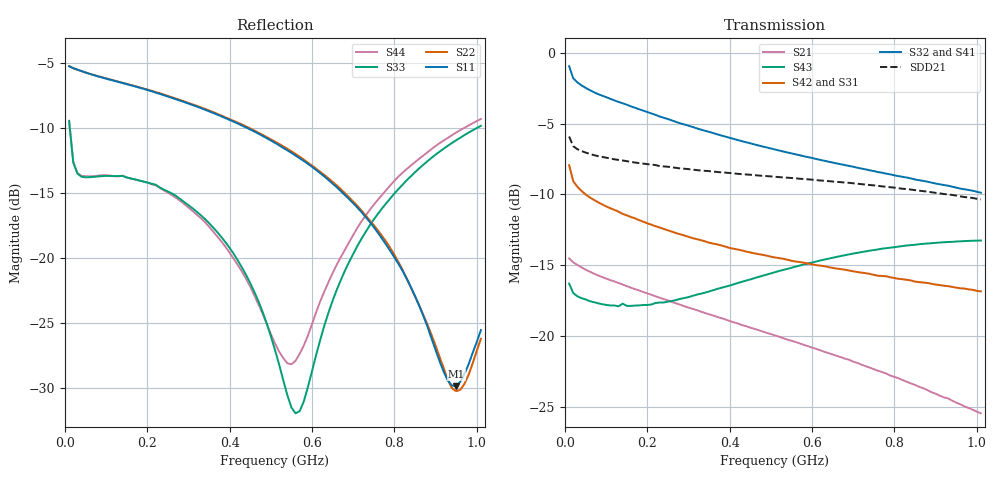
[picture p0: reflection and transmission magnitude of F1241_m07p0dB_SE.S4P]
! Integrated Device Technology
! Corporate Headquarters
! 6024 Silver Creek Valley Road
! San Jose, CA 95138  USA
! Phone:  1-408-284-8200
! Toll Free:  1-800-223-1366
! Webpage:  http://www.idt.com/
! Timing and RF Division
! 515 Groton Road, Suite 102
! Westford, MA 01886-6024
! Device:  F1241
! Description: Dual Intermediate Frequency Digital Variable Gain Amplifier
! Frequency:  10.0 -  500.00 MHz
! Package:  5x5 mm QFN Plastic Package: 32 pin
! Ports:  8 RF, 20 DC
!  Pin  1  = GA3  Pin 17  = RF OUT_B+
!  Pin  2  = GA4  Pin 18  = RF OUT_B-
!  Pin  3  = GA5  Pin 19  = STBY_B
!  Pin  4  = ISET_A  Pin 20  = Ground
!  Pin  5  = ISET_B  Pin 21  = Ground
!  Pin  6  = GB5  Pin 22  = STB_A
!  Pin  7  = GB4  Pin 23  = RF OUT_A-  = Port 4
!  Pin  8  = GB3  Pin 24  = RF OUT_A+  = Port 3
!  Pin  9  = GB2  Pin 25  = NO CONNECT
!  Pin 10  = GB1  Pin 26  = NO CONNECT
!  Pin 11  = RF IN_B+  Pin 27  = VCC
!  Pin 12  = RF IN_B-  Pin 28  = Ground
!  Pin 13  = Ground  Pin 29  = RF IN_A-  = Port 2
!  Pin 14  = VCC  Pin 30  = RF IN_A+  = Port 1
!  Pin 15  = NO CONNECT  Pin 31  = GA1
!  Pin 16  = NO CONNECT  Pin 32  = GA2
! State:  27
! Gain State:  -7.0 dB
! Voltages:  Vcc = +5.00 Volts  Icc approximately 160.0 mA or 80 mA per channel.
! Data:  The device was measured on a custom evaluation board which has
!  individual transmission lines to the RF pins.  Data was collected
!  using a calibrated network analyzer.  The evaluation board was
!  de-embedded using a port reference technique.
!  The reference plane is the edge of the package pin.
!  Only Channel A was measured.
!  This data is in single-ended operation.  If your needs are balanced
!  or differential S-parameters then this file needs to be used a
!  linear simulator.
! Misc:  Lot Code  160028MY
!  Action Tracker AT004
! Date Measured:  2014-08-14
! Date:  2014-08-28  MJV
! Note:
!  Integrated Device Technology supplies this data as a sample of measured
!  data at the package pin for this product.  Your particular data for this
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# Hz S dB R 50
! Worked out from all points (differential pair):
!   101 points, 10 MHz to 1.01 GHz, reference 50 ohm
!   strongest paths, dB at 10 MHz, 260 MHz, 510 MHz, 760 MHz, 1.01 GHz:
!     S32: -0.9, -4.8, -6.8, -8.4, -9.9
!     S41: -0.9, -4.8, -6.9, -8.6, -10.2
!     S42: -7.9, -12.6, -14.4, -15.7, -16.8
!     S31: -7.9, -12.7, -14.5, -15.8, -16.9
!     S43: -16.3, -17.5, -15.5, -13.9, -13.2
!     S21: -14.5, -17.6, -19.9, -22.4, -25.4
!   taken as a pair (ports 2,1 in; 3,4 out), SDD21 dB: -5.9, -8.1, -8.8, -9.4, -10.4
!   lowest |S11| = -29.9 dB at 950 MHz (marker M1), VSWR 1.07, Z = 51.9 + j2.67 ohm
!   |S11| at or under -10 dB: 441.9 MHz to end of sweep
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1e7  -5.26 -4.8  -14.50 -9.3  -33.43 -2.3  -25.85 6.0
     -14.51 -9.3  -5.25 -4.7  -25.88 5.7  -33.45 -2.4
     -7.94 157.2  -0.95 166.1  -9.50 -43.8  -16.34 177.9
     -0.91 166.2  -7.93 157.3  -16.29 178.0  -9.45 -43.6
4e7  -5.63 -6.3  -15.13 -11.0  -34.22 -7.8  -26.17 -4.7
     -15.14 -11.1  -5.64 -6.1  -26.18 -4.4  -34.20 -7.8
     -9.76 156.7  -2.30 165.3  -13.76 -14.2  -17.37 167.9
     -2.26 165.1  -9.75 156.6  -17.31 167.9  -13.70 -13.8
3.9e8  -9.25 -19.5  -18.80 -38.0  -36.58 -6.2  -27.80 -19.7
       -18.82 -38.2  -9.20 -18.1  -27.60 -19.3  -36.57 -8.1
       -13.77 77.5  -5.92 120.0  -18.81 -12.2  -16.59 107.0
       -5.99 118.7  -13.69 76.7  -16.50 106.6  -19.16 -7.1
5.6e8  -12.13 -22.2  -20.38 -45.6  -35.97 -3.4  -27.80 -25.1
       -20.41 -45.8  -12.01 -20.4  -27.44 -25.4  -36.00 -5.5
       -14.84 49.1  -7.17 103.5  -31.96 53.5  -15.21 83.2
       -7.30 102.0  -14.73 47.7  -15.09 83.0  -27.91 68.2
7.2e8  -16.48 -21.6  -21.94 -51.3  -35.10 -4.2  -27.85 -32.2
       -22.01 -51.6  -16.36 -20.1  -27.23 -32.8  -35.10 -6.9
       -15.65 26.5  -8.17 89.1  -18.54 126.5  -14.21 62.6
       -8.38 87.6  -15.52 24.2  -14.07 62.4  -17.20 120.1
9.5e8  -29.87 53.2  -24.56 -55.9  -33.64 -9.2  -28.02 -42.6
       -24.68 -56.1  -30.26 53.5  -27.15 -44.2  -33.68 -12.1
       -16.68 -0.3  -9.52 69.2  -10.95 123.8  -13.48 36.5
       -9.80 68.3  -16.57 -3.9  -13.32 36.4  -10.36 120.1
1.01e9  -25.56 100.0  -25.32 -56.1  -33.32 -11.8  -28.11 -45.2
        -25.44 -56.0  -26.23 100.8  -27.17 -47.3  -33.34 -14.6
        -16.93 -6.2  -9.88 64.4  -9.84 122.2  -13.40 30.4
        -10.17 63.5  -16.84 -10.0  -13.25 30.4  -9.32 118.5
